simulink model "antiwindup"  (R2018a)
settings: Solver=FixedStepAuto  StartTime=0.0  StopTime=20  FixedStep=0.01  RelTol=1e-3

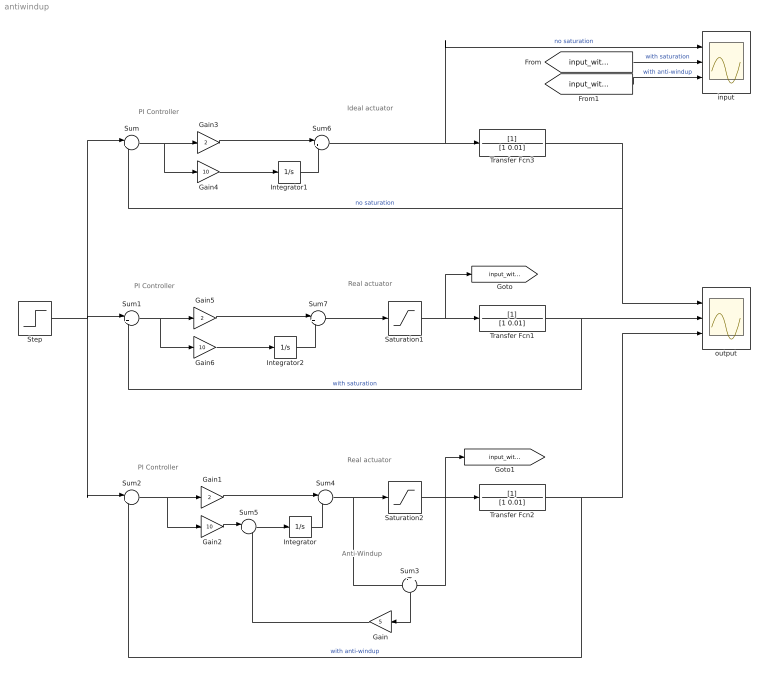
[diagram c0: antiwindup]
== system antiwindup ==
  note: Ideal actuator
  note: Real actuator
  note: Anti-Windup
  note: PI Controller
  note: PI Controller
  note: PI Controller
  note: Real actuator
  Gain : Gain  Gain=5
  Gain1 : Gain  Gain=2
  Gain2 : Gain  Gain=10
  Gain3 : Gain  Gain=2
  Gain4 : Gain  Gain=10
  Gain5 : Gain  Gain=2
  Gain6 : Gain  Gain=10
  Integrator : Integrator
  Integrator1 : Integrator
  Integrator2 : Integrator
  Saturation1 : Saturate
  Saturation2 : Saturate
  Step : Step  SampleTime=0
  Sum : Sum  Inputs=|+-
  Sum1 : Sum  Inputs=|+-
  Sum2 : Sum  Inputs=|+-
  Sum3 : Sum  Inputs=-|+
  Sum{4..7} (4 alike) : Sum  Inputs=|++
  Transfer Fcn1 : TransferFcn  Denominator=[1 0.01]
  Transfer Fcn2 : TransferFcn  Denominator=[1 0.01]
  Transfer Fcn3 : TransferFcn  Denominator=[1 0.01]
  input : Scope  NumInputPorts=3
  output : Scope  NumInputPorts=3
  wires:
  Sum6/1 -> input/1, Transfer Fcn3/1  "no saturation"
  Sum/1 -> Gain4/1, Gain3/1
  Transfer Fcn3/1 -> Sum/2, output/1  "no saturation"
  Transfer Fcn1/1 -> Sum1/2, output/2  "with saturation"
  Sum1/1 -> Gain6/1, Gain5/1
  Saturation1/1 -> [input_with_sat], Transfer Fcn1/1
  Step/1 -> Sum2/1, Sum1/1, Sum/1
  Sum4/1 -> Saturation2/1, Sum3/1
  Sum2/1 -> Gain1/1, Gain2/1
  Saturation2/1 -> [input_with_antiwindup], Sum3/2, Transfer Fcn2/1
  Transfer Fcn2/1 -> Sum2/2, output/3  "with anti-windup"
  Sum3/1 -> Gain/1
  Gain1/1 -> Sum4/1
  Gain2/1 -> Sum5/1
  Integrator/1 -> Sum4/2
  Gain/1 -> Sum5/2
  Sum5/1 -> Integrator/1
  Gain4/1 -> Integrator1/1
  Integrator1/1 -> Sum6/2
  Gain3/1 -> Sum6/1
  Gain5/1 -> Sum7/1
  Integrator2/1 -> Sum7/2
  Gain6/1 -> Integrator2/1
  Sum7/1 -> Saturation1/1
  [input_with_sat] -> input/2  "with saturation"
  [input_with_antiwindup] -> input/3  "with anti-windup"
